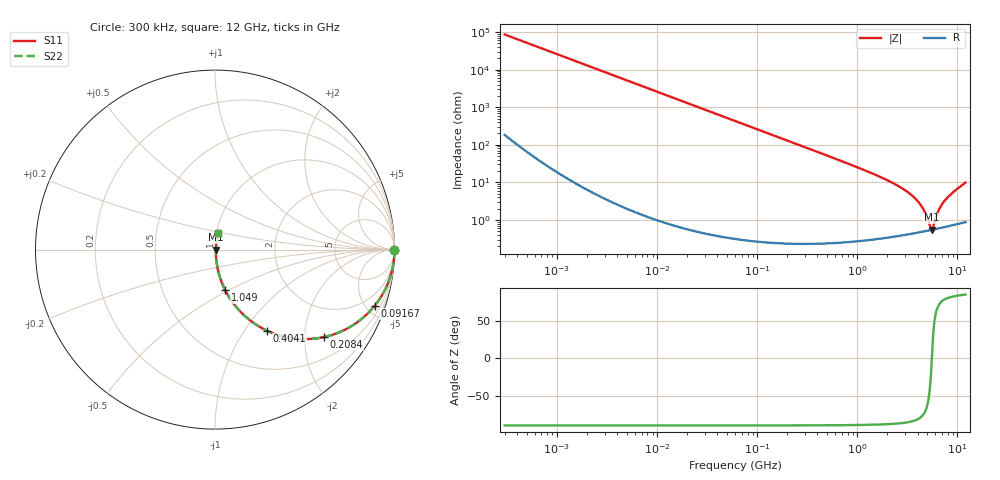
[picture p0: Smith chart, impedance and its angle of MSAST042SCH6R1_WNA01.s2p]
! MSAST042SCH6R1_WNA01  S-PARAMETER MODEL  ( General Type )
! Model Generated by TAIYO YUDEN Corporation (http://www.ty-top.com)
! Version 1.0
! TAIYO YUDEN Control No. 150820
! Copyright(c) 2015 TAIYO YUDEN CO.,LTD. All Rights Reserved.
! Product Description (link to TY-COMPAS)
! https://ds.yuden.co.jp/TYCOMPAS/or/detail?pn=MSAST042SCH6R1BWNA01&u=M
! Products Name : Multilayer Ceramic Capacitors
! Characteristics :
!  Capacitance : 6.1 pF , Rated Voltage : 25V , TCC : CH / C0H
!  Case Size : 0.4 x 0.2 / 0.016 x 0.008 [mm/inch] , Thickness : 0.2 / 0.008 [mm/inch]
!  (Conditions: Temperature = 25 degC , DC Bias Current/Voltage = 0A / 0V)
! External Node Assignments :
!  1  o---| |---o  2
! GND o---------o GND
! Frequency Range : 0.3MHz  -  12000MHz  [ 401 STEP ]
# MHz S RI R 50
! Freq[MHz].  S11 Real  S11 Imag  S21 Real  S21 Imag  S12 Real  S12 Imag  S22 Real  S22 Imag
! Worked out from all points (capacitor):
!   401 points, 300 kHz to 12 GHz, reference 50 ohm
!   read as one part in series: C = 6.13 pF near 316.3 kHz
!   lowest |Z| = 544 mohm at 5.566 GHz (marker M1)
!   series resonance near 5.555 GHz, so ESL is about 130 pH
!   S11 on the Smith chart (normalised r, x): 300 kHz: open; 91.67 MHz: 1.01, -5.67; 208.4 MHz: 1.00, -2.49; 404.1 MHz: 1.00, -1.28; 1.049 GHz: 1.01, -0.48; 12 GHz: 1.02, +0.20
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0.3  1 -0.00115  3.79e-06 0.00115  3.79e-06 0.00115  1 -0.00115
1.769972  1 -0.00681  4.99e-05 0.00681  4.99e-05 0.00681  1 -0.00681
10.44266  0.9984 -0.0401  0.00163 0.0401  0.00163 0.0401  0.9984 -0.0401
27.82928  0.9886 -0.1059  0.0114 0.1059  0.0114 0.1059  0.9886 -0.1059
60  0.9492 -0.2192  0.0508 0.2192  0.0508 0.2192  0.9492 -0.2192
91.67136  0.889 -0.3137  0.111 0.3137  0.111 0.3137  0.889 -0.3137
208.3979  0.6075 -0.4874  0.3925 0.4874  0.3925 0.4874  0.6075 -0.4874
353.9943  0.3486 -0.475  0.6514 0.475  0.6514 0.475  0.3486 -0.475
404.1309  0.2909 -0.4524  0.7091 0.4524  0.7091 0.4524  0.2909 -0.4524
634.0297  0.142 -0.3461  0.858 0.3461  0.858 0.3461  0.142 -0.3461
1048.836  0.0563 -0.2248  0.9437 0.2248  0.9437 0.2248  0.0563 -0.2248
2088.533  0.0146 -0.1049  0.9854 0.1049  0.9854 0.1049  0.0146 -0.1049
3026.31  0.00758 -0.0598  0.9924 0.0598  0.9924 0.0598  0.00758 -0.0598
3841.137  0.00569 -0.0351  0.9943 0.0351  0.9943 0.0351  0.00569 -0.0351
4502.883  0.00522 -0.0197  0.9948 0.0197  0.9948 0.0197  0.00522 -0.0197
5278.635  0.00528 -0.00491  0.9947 0.00491  0.9947 0.00491  0.00528 -0.00491
5565.855  0.00541 0.000196  0.9946 -0.000196  0.9946 -0.000196  0.00541 0.000196
5868.704  0.00561 0.00615  0.9944 -0.00615  0.9944 -0.00615  0.00561 0.00615
6524.734  0.00622 0.0174  0.9938 -0.0174  0.9938 -0.0174  0.00622 0.0174
7254.098  0.00712 0.0287  0.9929 -0.0287  0.9929 -0.0287  0.00712 0.0287
9207.246  0.0104 0.0552  0.9896 -0.0552  0.9896 -0.0552  0.0104 0.0552
12000  0.0178 0.0951  0.9822 -0.0951  0.9822 -0.0951  0.0178 0.0951
